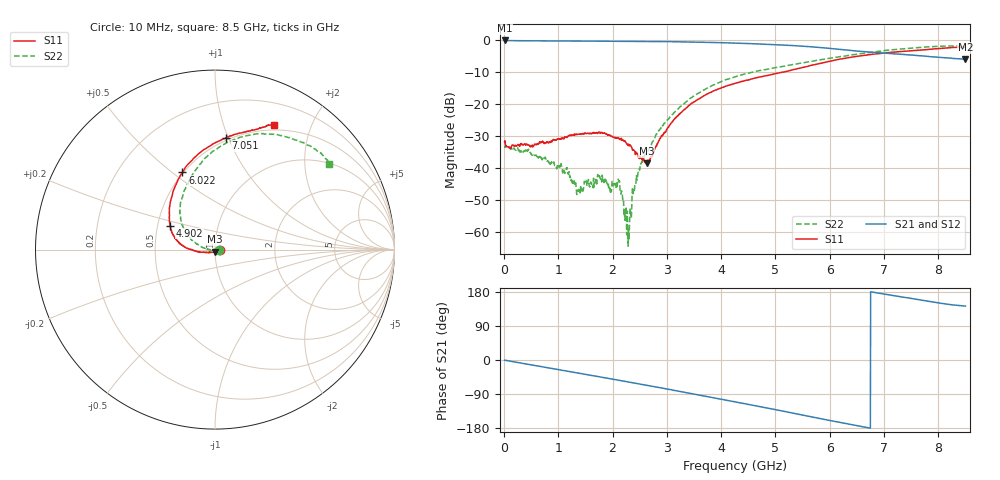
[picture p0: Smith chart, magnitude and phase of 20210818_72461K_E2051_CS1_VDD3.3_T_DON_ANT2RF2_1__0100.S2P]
!Agilent Technologies,E5071C,MY46417908,A.11.23
!Date: Wed Aug 18 14:26:19 2021
!Data & Calibration Information:
!Freq	S11:SOLT2(ON)	S21:SOLT2(ON)	S12:SOLT2(ON)	S22:SOLT2(ON)
!PortZ  Port1:50+j0  Port2:50+j0
!Above PortZ is port z conversion or system Z0 setting when saving the data.
!When reading, reference impedance value at option line is always used.
# Hz S dB R 50
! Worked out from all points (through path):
!   1601 points, 10 MHz to 8.5 GHz, reference 50 ohm
!   highest |S21| = -0.24 dB at 10 MHz (marker M1); lowest = -6.1 dB at 8.5 GHz (marker M2)
!   group delay of S21, straight-line fit = 73.7 ps
!   lowest |S11| = -38.5 dB at 2.631 GHz (marker M3), VSWR 1.02, Z = 50 - j1.19 ohm
!   |S11| at or under -10 dB: start of sweep to 5.17 GHz
!   |S22| runs from -64.4 to -1.9 dB; largest |S21 - S12| = 0.0032
!   S11 on the Smith chart (normalised r, x): 10 MHz: 1.05, +0.00; 4.902 GHz: 0.58, +0.17; 6.022 GHz: 0.49, +0.54; 7.051 GHz: 0.48, +0.98; 8.5 GHz: 0.45, +1.49
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1e7  -31.82 0.9  -0.24 -0.4  -0.24 -0.4  -33.32 -9.2
5.087875e8  -33.19 -20.2  -0.35 -13.0  -0.35 -13.0  -35.76 -34.3
1.023494e9  -31.03 -14.4  -0.38 -25.9  -0.38 -25.9  -39.22 -38.3
1.426769e9  -29.48 -7.5  -0.43 -36.1  -0.43 -36.1  -47.36 -4.4
1.766369e9  -29.09 -5.4  -0.46 -44.6  -0.46 -44.6  -42.83 33.4
1.941475e9  -29.72 -10.5  -0.47 -49.1  -0.48 -49.1  -46.83 24.5
2.09005e9  -30.58 -9.8  -0.49 -52.8  -0.49 -52.8  -44.61 24.7
2.143112e9  -30.87 -12.5  -0.49 -54.1  -0.49 -54.1  -47.29 22.2
2.265156e9  -32.60 -19.8  -0.51 -57.3  -0.51 -57.3  -56.19 60.0
2.3023e9  -33.08 -23.2  -0.51 -58.2  -0.51 -58.2  -62.38 -172.2
2.403119e9  -34.69 -32.0  -0.53 -60.8  -0.53 -60.8  -46.70 -159.6
2.519856e9  -36.89 -55.8  -0.54 -63.8  -0.55 -63.8  -38.75 -168.9
2.631288e9  -38.48 -87.4  -0.54 -66.8  -0.54 -66.8  -35.32 -172.5
2.843538e9  -31.77 -143.5  -0.58 -72.4  -0.58 -72.4  -28.52 179.0
3.437838e9  -20.10 -173.4  -0.71 -88.2  -0.71 -88.2  -18.18 160.1
4.255e9  -13.65 168.3  -1.06 -110.4  -1.06 -110.4  -11.59 136.9
4.902362e9  -10.95 151.8  -1.48 -128.2  -1.49 -128.2  -9.04 120.4
5.671769e9  -7.97 125.6  -2.23 -150.3  -2.25 -150.3  -6.72 103.0
6.021981e9  -6.62 112.9  -2.74 -160.3  -2.75 -160.4  -5.73 95.5
7.051394e9  -4.07 84.4  -4.22 172.8  -4.23 172.7  -3.31 70.5
7.088538e9  -4.01 83.8  -4.27 171.9  -4.28 171.8  -3.26 69.7
8.5e9  -2.32 64.5  -6.14 142.3  -6.09 142.2  -2.02 36.8
